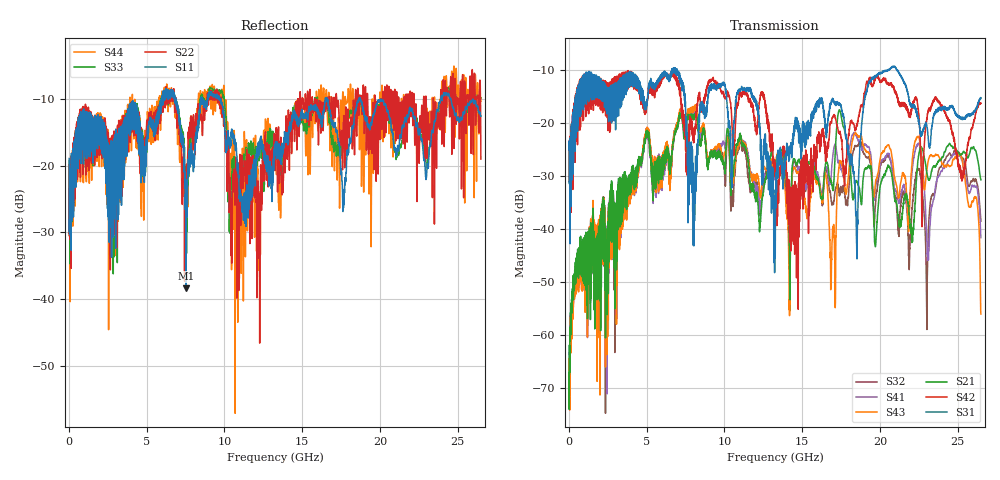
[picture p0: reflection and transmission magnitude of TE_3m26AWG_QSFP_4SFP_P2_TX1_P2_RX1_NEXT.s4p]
!Agilent Technologies,N5222A,MY51421691,A.10.00.00
!Agilent N5222A: A.10.00.00
!Date: Friday, January 30, 2015 12:35:06
!Correction: S11(Full 4 Port(1,2,3,4))
!S12(Full 4 Port(1,2,3,4))
!S13(Full 4 Port(1,2,3,4))
!S14(Full 4 Port(1,2,3,4))
!S21(Full 4 Port(1,2,3,4))
!S22(Full 4 Port(1,2,3,4))
!S23(Full 4 Port(1,2,3,4))
!S24(Full 4 Port(1,2,3,4))
!S31(Full 4 Port(1,2,3,4))
!S32(Full 4 Port(1,2,3,4))
!S33(Full 4 Port(1,2,3,4))
!S34(Full 4 Port(1,2,3,4))
!S41(Full 4 Port(1,2,3,4))
!S42(Full 4 Port(1,2,3,4))
!S43(Full 4 Port(1,2,3,4))
!S44(Full 4 Port(1,2,3,4))
!S4P File: Measurements: <S11,S12,S13,S14>,
!<S21,S22,S23,S24>,
!<S31,S32,S33,S34>,
!<S41,S42,S43,S44>:
# Hz S  dB  R 50.0
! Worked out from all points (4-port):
!   2650 points, 10 MHz to 26.5 GHz, reference 50 ohm
!   strongest paths, dB at 10 MHz, 6.63 GHz, 13.26 GHz, 19.88 GHz, 26.5 GHz:
!     S31: -25.0, -10.3, -36.3, -10.8, -15.2
!     S42: -24.9, -11.2, -27.5, -11.3, -16.3
!     S21: -67.0, -25.5, -27.6, -36.1, -30.7
!     S43: -67.4, -25.8, -27.8, -29.4, -56.0
!     S41: -70.3, -26.2, -30.0, -29.9, -41.6
!     S32: -69.3, -25.2, -28.0, -31.1, -38.5
!   lowest |S11| = -38.4 dB at 7.52 GHz (marker M1), VSWR 1.02, Z = 51.2 + j0.169 ohm
!   |S11| at or under -10 dB: start of sweep to 5.956 GHz; 9.721 GHz to 16.5 GHz (6.776 GHz wide, 51.7 % of centre); 18.73 GHz to 23.92 GHz (5.185 GHz wide, 24.3 % of centre)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
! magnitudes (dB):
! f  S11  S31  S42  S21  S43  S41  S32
! 10 MHz  -18.9  -25.0  -24.9  -67.0  -67.4  -70.3  -69.3
! 7.52 GHz  -38.4  -19.8  -23.2  -20.1  -19.5  -19.9  -19.8
! 14.13 GHz  -15.1  -26.5  -31.1  -37.8  -44.4  -37.7  -42.0
! 18.5 GHz  -11.0  -42.3  -20.4  -30.8  -22.2  -22.6  -24.4
! 19.82 GHz  -10.6  -11.0  -11.2  -38.6  -30.3  -30.5  -32.8
! 25.14 GHz  -13.3  -18.9  -28.0  -25.9  -25.8  -26.1  -25.9
! 26.5 GHz  -12.6  -15.2  -16.3  -30.7  -56.0  -41.6  -38.5
